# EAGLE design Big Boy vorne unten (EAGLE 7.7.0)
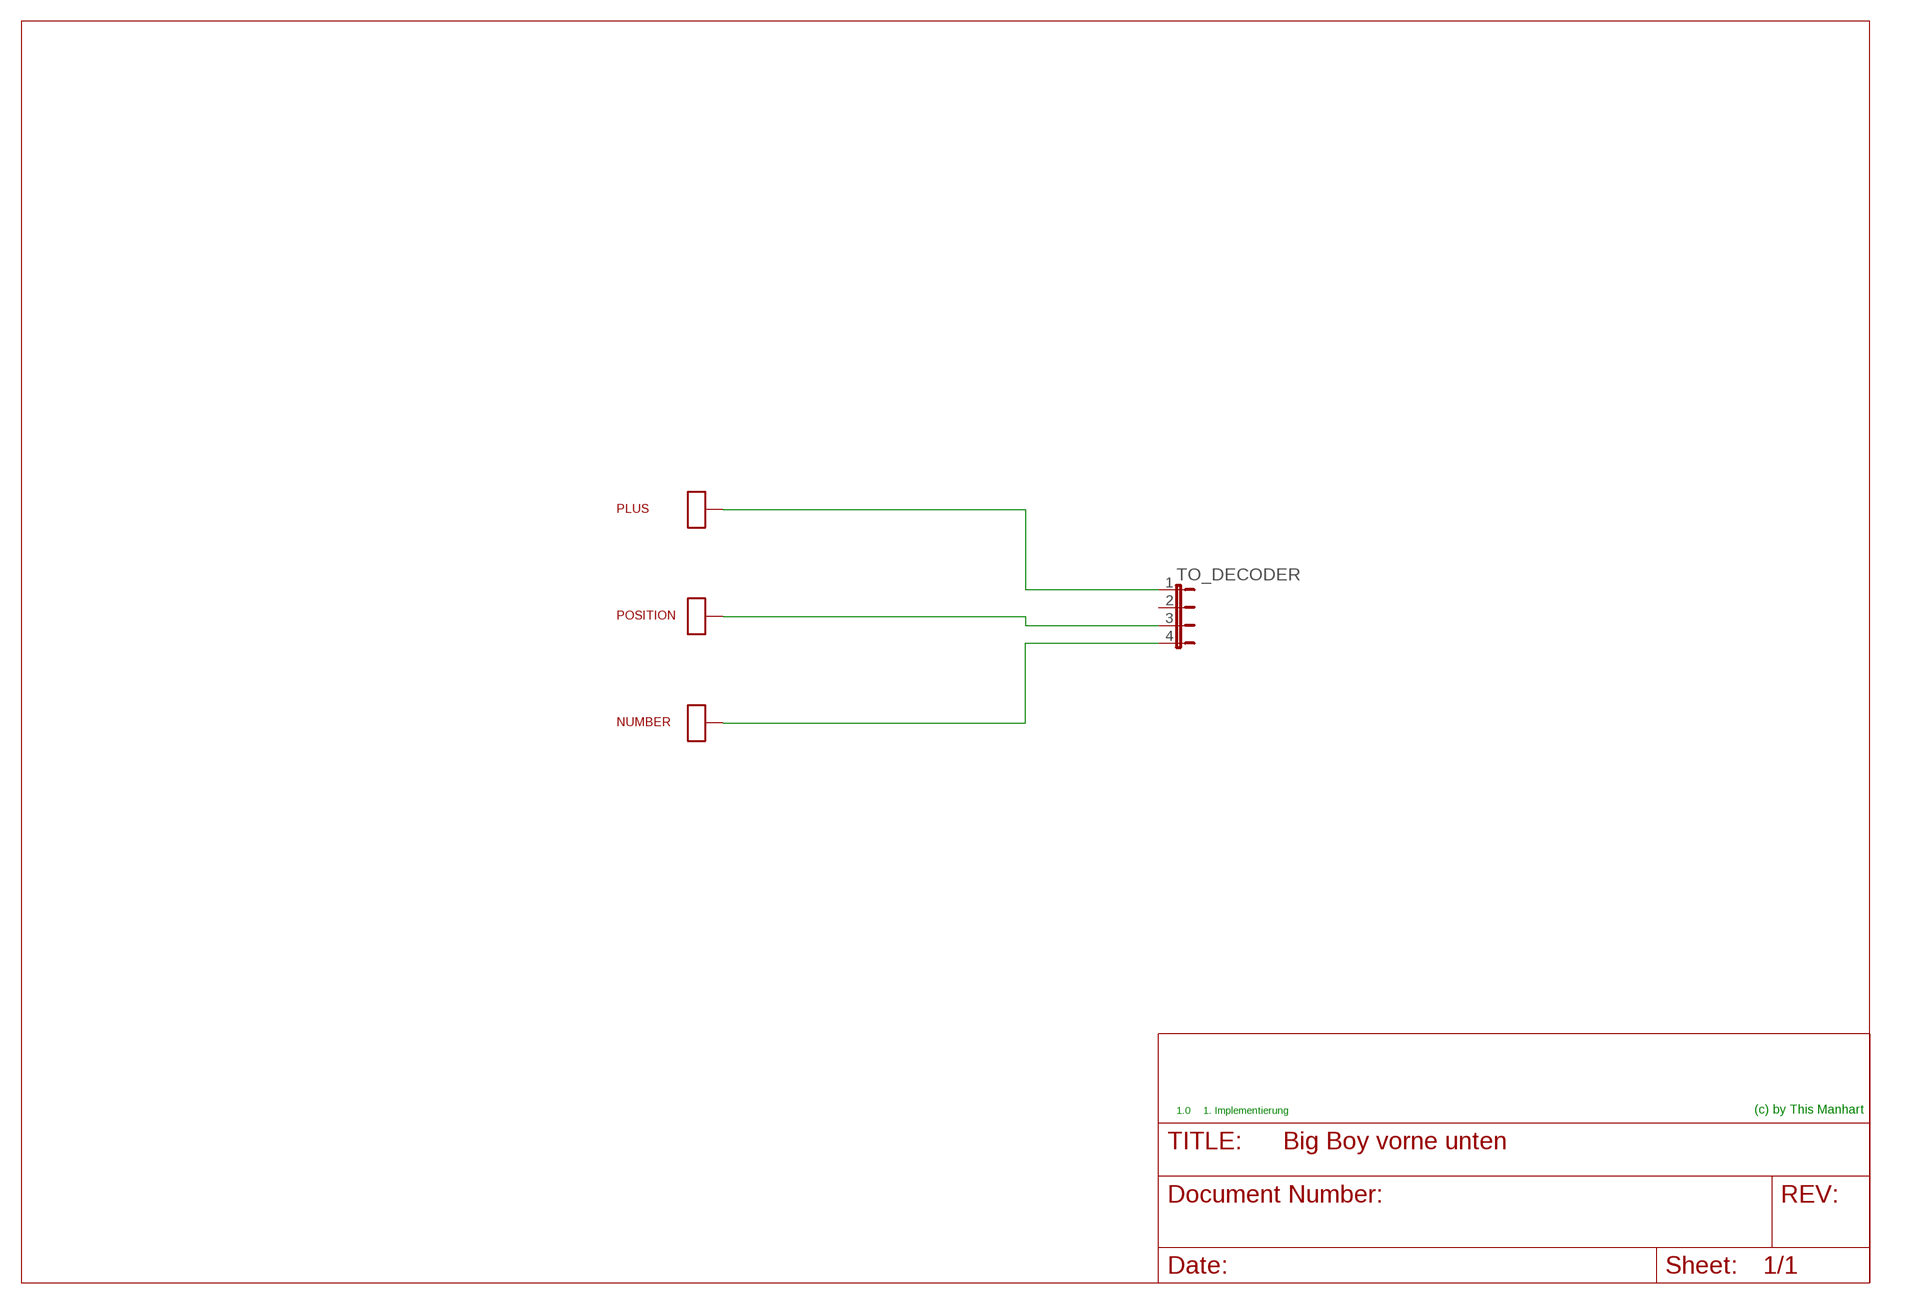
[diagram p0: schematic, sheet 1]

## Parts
NUMBER  SMD_LOETPAD  [SMD_LOETPAD_XL]
PLUS  SMD_LOETPAD  [SMD_LOETPAD_XL]
POSITION  SMD_LOETPAD  [SMD_LOETPAD_XL]
TO_DECODER  JUMPER_4P  [JUMPER_4P_2.54_OHNE]

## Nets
N$1: PLUS.P$1 TO_DECODER.1
N$2: POSITION.P$1 TO_DECODER.3
N$3: NUMBER.P$1 TO_DECODER.4
Unconnected: TO_DECODER.2

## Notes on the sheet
- 1.0 | 1. Implementierung | (c) by This Manhart

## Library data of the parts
NUMBER PLUS POSITION = 0_mm:SMD_LOETPAD
TO_DECODER = 0_mm:JUMPER_4P

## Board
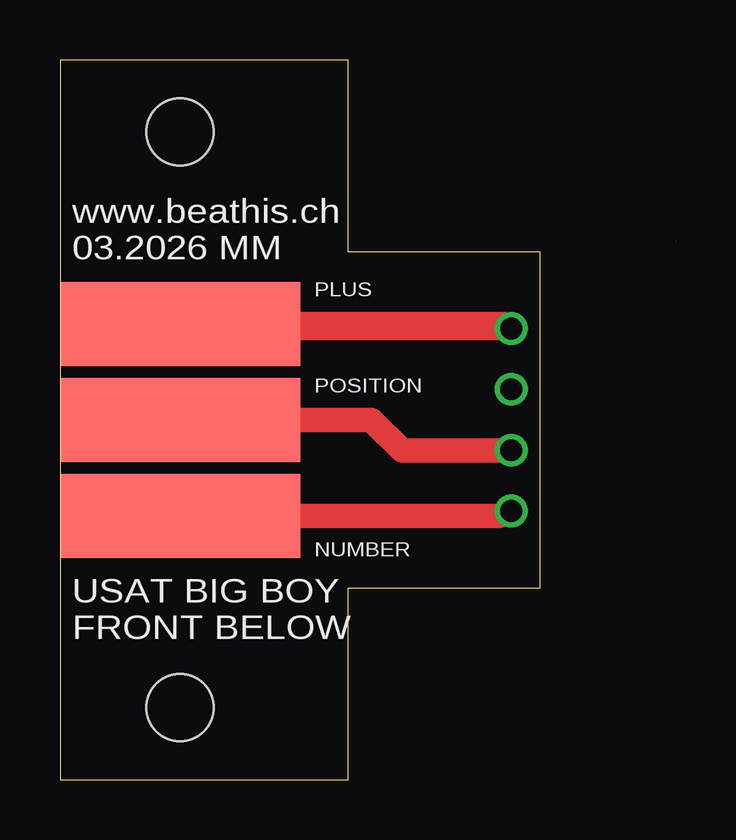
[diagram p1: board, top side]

Size 25.66 x 30 mm. Coordinates in mm from the lower left corner, seen from the top.
Outline: 25.65,22.45 25.66,22.45
Outline: 20,8 20,22 12,22 12,30 0,30 0,0 12,0 12,8 20,8
Copper layers (1*16): Top 0.035mm / dielectric 1.5mm / Bottom 0.035mm
Design rules "pcb-pool": minimum track width 6mil, minimum drill 12mil, track to track 6mil, track to pad 6mil, pad to pad 6mil, via to via 6mil, smd to smd 8mil, copper to edge 40mil, drill to drill 20mil, minimum pad ring 8mil, minimum via ring 8mil, stop-mask expansion 6mil, vias tented up to drill 0mil, thermal gap 10mil
Holes 2.8 mm at 5,3 5,27

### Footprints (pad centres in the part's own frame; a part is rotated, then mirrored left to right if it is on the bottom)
SMD_LOETPAD_XL = smd 10 x 3.5: P$1 0,0
JUMPER_4P_2.54_OHNE = drill 0.914: 1 -3.81,0; 2 -1.27,0; 3 1.27,0; 4 3.81,0

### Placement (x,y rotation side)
NUMBER  5,11 0 top
PLUS  5,19 180 top
POSITION  5,15 0 top
TO_DECODER  18.8,15 270 top

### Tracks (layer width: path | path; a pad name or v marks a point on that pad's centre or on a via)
N$1
  Top 1.016: PLUS.P$1 18.5,19 TO_DECODER.1
N$2
  Top 1.016: POSITION.P$1 12.96,15 14.25,13.71 18.48,13.71 TO_DECODER.3
N$3
  Top 1.016: NUMBER.P$1 18.31,11 TO_DECODER.4
N$4
  Top 1.016: 18.39,18.82 5.02,18.82 5.02,18.93

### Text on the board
tNames: www.beathis.ch / 03.2026 MM | PLUS | POSITION | NUMBER | USAT BIG BOY / FRONT BELOW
